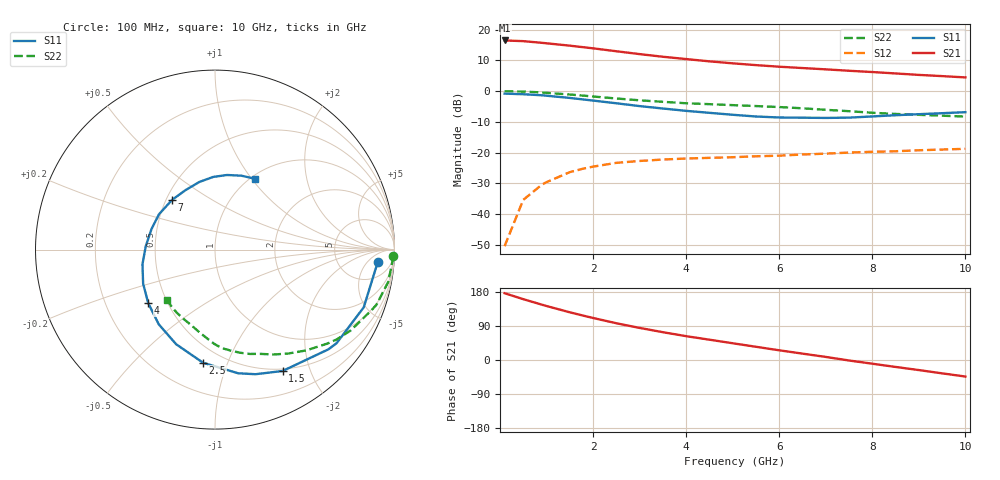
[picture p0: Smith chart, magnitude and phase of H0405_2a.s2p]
!HBFP-0405
!S-PARAMETERS at Vce=2V  Ic=2mA.  LAST UPDATED 05-29-98
# ghz s ma r 50
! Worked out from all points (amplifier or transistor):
!   23 points, 100 MHz to 10 GHz, reference 50 ohm
!   highest |S21| = 16.5 dB at 100 MHz (marker M1)
!   |S21| within 3 dB of that: start of sweep to 2.232 GHz
!   unconditionally stable (mu >= 1): 4.358 GHz to end of sweep
!   at 1 GHz: K = 0.13, MSG = 22.6 dB, |S12| = -29.6 dB
!   at 4.5 GHz: K = 1.03, MAG = 14.6 dB, |S12| = -21.7 dB
!   at 10 GHz: K = 1.68, MAG = 6.8 dB, |S12| = -18.8 dB
!   lowest NFmin = 1.07 dB at 900 MHz
!   S11 on the Smith chart (normalised r, x): 100 MHz: 13, -10; 1.5 GHz: 0.47, -1.60; 2.5 GHz: 0.39, -0.82; 4 GHz: 0.39, -0.30; 7 GHz: 0.54, +0.34; 10 GHz: 1.05, +1.04
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0.1  0.91 -4.2  6.665 176.2  0.003 88.5  0.995 -2.2
0.5  0.889 -21.2  6.496 160.6  0.017 80.5  0.982 -10.5
0.9  0.855 -37.6  6.101 146.0  0.03 71.9  0.951 -18.8
1  0.841 -41.4  5.993 142.5  0.033 69.6  0.937 -20.9
1.5  0.774 -60.9  5.484 125.9  0.048 57.5  0.88 -30.8
1.8  0.73 -72.0  5.164 116.8  0.055 50.6  0.843 -36.4
2  0.701 -79.4  4.964 110.9  0.059 46.4  0.817 -39.8
2.5  0.634 -96.0  4.45 97.0  0.068 37.0  0.758 -47.8
3  0.57 -112.3  3.996 84.7  0.073 28.7  0.708 -54.9
3.5  0.521 -127.0  3.62 73.4  0.077 21.7  0.669 -60.9
4  0.477 -141.2  3.32 62.9  0.08 15.6  0.634 -66.4
4.5  0.443 -154.7  3.047 53.6  0.082 10.7  0.613 -71.5
5  0.412 -168.7  2.829 44.2  0.084 6.0  0.591 -76.4
5.5  0.386 177.1  2.646 34.9  0.087 1.6  0.571 -80.8
6  0.372 162.2  2.493 25.6  0.089 -2.1  0.55 -86.1
6.5  0.369 147.7  2.371 16.8  0.093 -7.0  0.525 -90.5
7  0.366 130.7  2.258 8.1  0.096 -10.7  0.496 -95.2
7.5  0.37 116.2  2.141 -1.3  0.1 -14.7  0.471 -100.2
8  0.387 102.9  2.042 -9.8  0.103 -19.2  0.444 -106.7
8.5  0.405 91.4  1.937 -18.3  0.105 -23.6  0.425 -113.9
9.5  0.437 70.5  1.753 -35.2  0.112 -32.4  0.398 -127.7
10  0.454 60.3  1.669 -43.7  0.115 -37.0  0.385 -133.5
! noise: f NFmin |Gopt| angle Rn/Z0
0.9  1.07  0.569  9.3  0.42
1.5  1.19  0.504  22  0.38
2  1.29  0.456  33.6  0.36
3  1.48  0.391  59.3  0.31
4  1.7  0.318  83.1  0.26
5.5  2  0.215  118.3  0.21
6.5  2.18  0.157  153.1  0.2
7.5  2.35  0.116  -154.8  0.24
8.5  2.65  0.163  -104.1  0.32
10  2.94  0.254  -61.4  0.53
